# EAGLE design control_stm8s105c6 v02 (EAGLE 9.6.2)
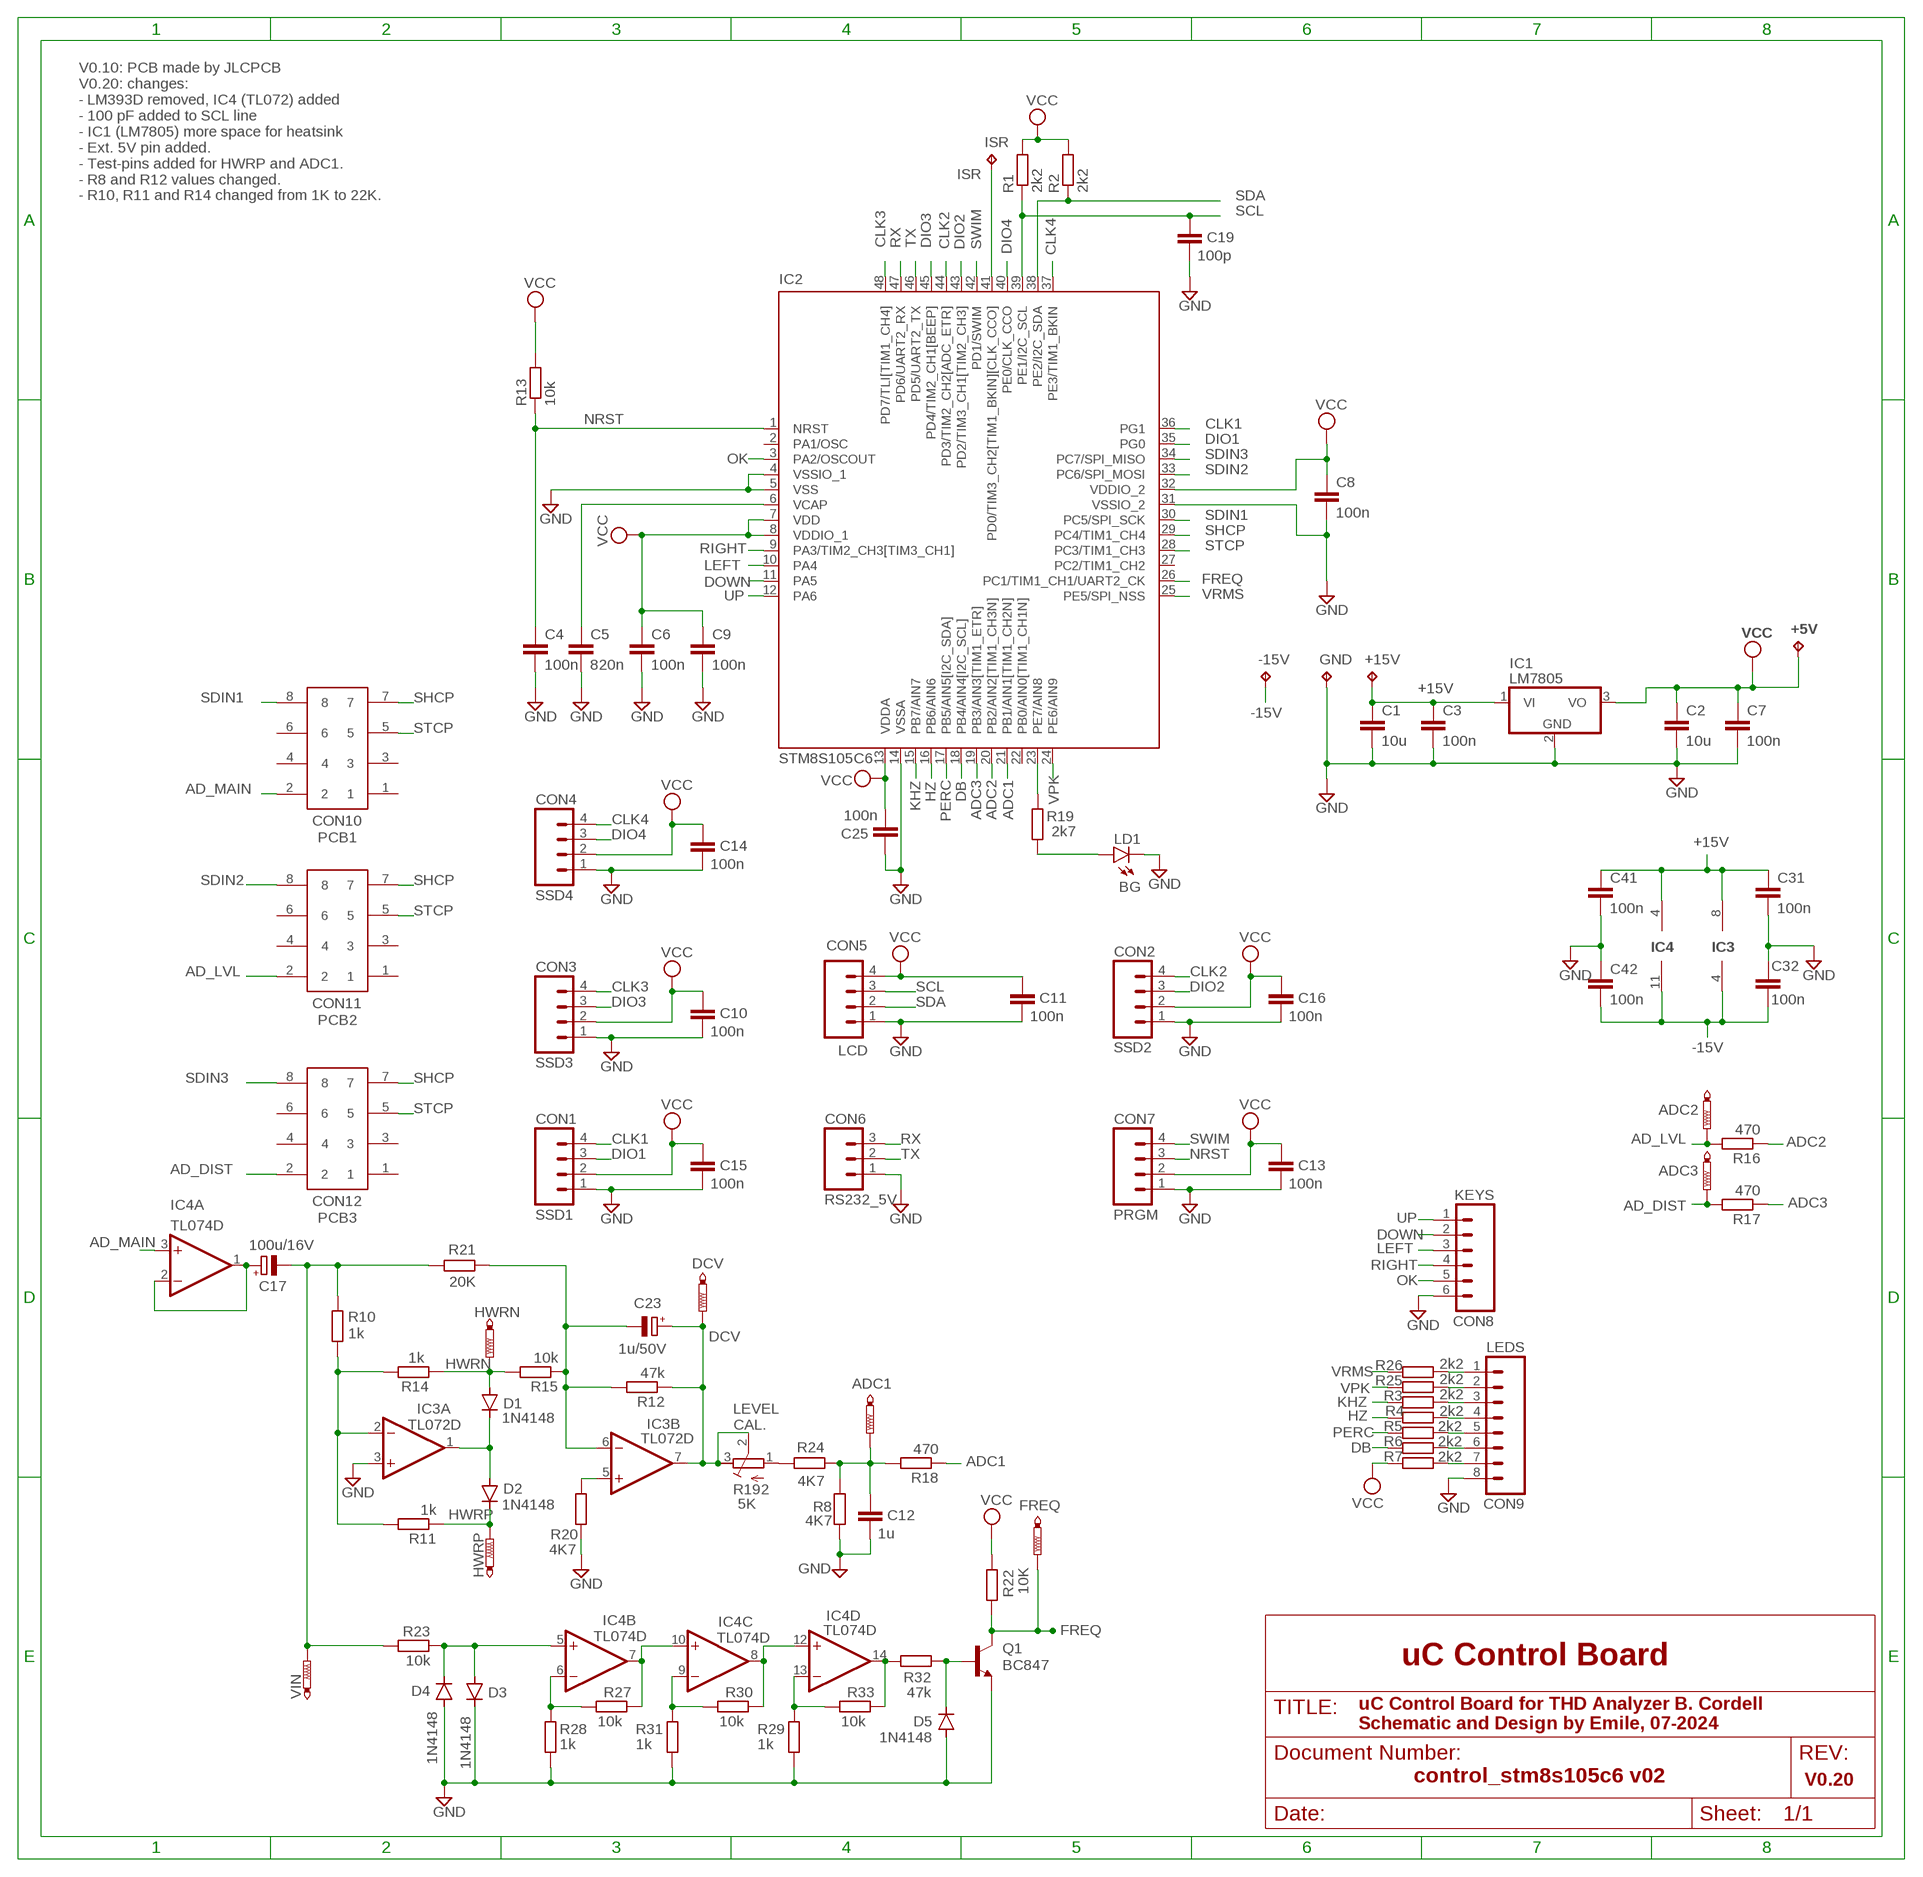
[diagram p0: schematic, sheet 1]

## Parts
+5V  TPPAD1-13Y  [P1-13Y]
+15V  TPPAD1-13Y  [P1-13Y]
-15V  TPPAD1-13Y  [P1-13Y]
ADC1  PTR1B2,54  [B2,54]
ADC2  PTR1B2,54  [B2,54]
ADC3  PTR1B2,54  [B2,54]
C1  10u  C-EUC1206  [C1206]
C2  10u  C-EUC1206  [C1206]
C3  100n  C-EUC1206  [C1206]
C4  100n  C-EUC1206K  [C1206K]
C5  820n  C-EUC1206K  [C1206K]
C6  100n  C-EUC1206K  [C1206K]
C7  100n  C-EUC1206  [C1206]
C8  100n  C-EUC1206K  [C1206K]
C9  100n  C-EUC1206K  [C1206K]
C10  100n  C-EUC1206  [C1206]
C11  100n  C-EUC1206  [C1206]
C12  1u  C-EUC1206  [C1206]
C13  100n  C-EUC1206  [C1206]
C14  100n  C-EUC1206  [C1206]
C15  100n  C-EUC1206  [C1206]
C16  100n  C-EUC1206  [C1206]
C17  100u/16V  CPOL-EUUD-6,3X8,8  [UD-6,3X5,8_NICHICON]
C19  100p  C-EUC1206  [C1206]
C23  1u/50V  CPOL-EUUD-4X5,8  [UD-4X5,8_NICHICON]
C25  100n  C-EUC1206  [C1206]
C31  100n  C-EUC1206  [C1206]
C32  100n  C-EUC1206  [C1206]
C41  100n  C-EUC1206  [C1206]
C42  100n  C-EUC1206  [C1206]
CON1  SSD1  M04  [04P]
CON2  SSD2  M04  [04P]
CON3  SSD3  M04  [04P]
CON4  SSD4  M04  [04P]
CON5  LCD  M04  [04P]
CON6  RS232_5V  M03  [03P]
CON7  PRGM  M04  [04P]
CON8  KEYS  M06  [06P]
CON9  LEDS  M08  [08P]
CON10  PCB1  61200821621  [61200821621]
CON11  PCB2  61200821621  [61200821621]
CON12  PCB3  61200821621  [61200821621]
D1  1N4148  D-SOD-80  [SOD80]
D2  1N4148  D-SOD-80  [SOD80]
D3  1N4148  D-SOD-80  [SOD80]
D4  1N4148  D-SOD-80  [SOD80]
D5  1N4148  D-SOD-80  [SOD80]
DCV  PTR1B2,54  [B2,54]
FREQ  PTR1B2,54  [B2,54]
GND  TPPAD1-13Y  [P1-13Y]
HWRN  PTR1B2,54  [B2,54]
HWRP  PTR1B2,54  [B2,54]
IC1  LM7805  7805TV  [TO220V]
IC2  STM8S105C6  STM8S105CV2  [LQFP48]
IC3  TL072D  [SO08]
IC4  TL074D  [SO14]
ISR  TPB2,54  [B2,54]
LD1  BG  LEDCHIPLED_1206  [CHIPLED_1206]
Q1  BC847  [SOT23]
R1  2k2  R-EU_R1206  [R1206]
R2  2k2  R-EU_R1206  [R1206]
R3  2k2  R-EU_M1206  [M1206]
R4  2k2  R-EU_M1206  [M1206]
R5  2k2  R-EU_M1206  [M1206]
R6  2k2  R-EU_M1206  [M1206]
R7  2k2  R-EU_M1206  [M1206]
R8  4K7  R-EU_R1206  [R1206]
R10  1k  R-EU_R1206  [R1206]
R11  1k  R-EU_R1206  [R1206]
R12  47k  R-EU_R1206  [R1206]
R13  10k  R-EU_R1206  [R1206]
R14  1k  R-EU_R1206  [R1206]
R15  10k  R-EU_R1206  [R1206]
R16  470  R-EU_R1206  [R1206]
R17  470  R-EU_R1206  [R1206]
R18  470  R-EU_R1206  [R1206]
R19  2k7  R-EU_M1206  [M1206]
R20  4K7  R-EU_R1206  [R1206]
R21  20K  R-EU_R1206  [R1206]
R22  10K  R-EU_R1206  [R1206]
R23  10k  R-EU_R1206  [R1206]
R24  4K7  R-EU_R1206  [R1206]
R25  2k2  R-EU_M1206  [M1206]
R26  2k2  R-EU_M1206  [M1206]
R27  10k  R-EU_R1206  [R1206]
R28  1k  R-EU_R1206  [R1206]
R29  1k  R-EU_R1206  [R1206]
R30  10k  R-EU_R1206  [R1206]
R31  1k  R-EU_R1206  [R1206]
R32  47k  R-EU_R1206  [R1206]
R33  10k  R-EU_R1206  [R1206]
R192  5K  R-TRIMM3296W  [RTRIM3296W]
VIN  PTR1B2,54  [B2,54]

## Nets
+15V: +15V.TP C1.1 C3.1 C31.1 C41.1 IC1.1(VI) IC3.8(P:V+) IC4.4(P:V+)
-15V: -15V.TP C32.2 C42.2 IC3.4(P:V-) IC4.11(P:V-)
AD_DIST: ADC3.TP CON12.2 R17.2
AD_LVL: ADC2.TP CON11.2 R16.2
AD_MAIN: CON10.2 IC4.3(A:+IN)
ADC1: IC2.21(PB1/AIN1[TIM1_CH2N]) R18.1
ADC2: IC2.20(PB2/AIN2[TIM1_CH3N]) R16.1
ADC3: IC2.19(PB3/AIN3[TIM1_ETR]) R17.1
CLK1: CON1.4 IC2.36(PG1)
CLK2: CON2.4 IC2.44(PD3/TIM2_CH2[ADC_ETR])
CLK3: CON3.4 IC2.48(PD7/TLI[TIM1_CH4])
CLK4: CON4.4 IC2.37(PE3/TIM1_BKIN)
DB: IC2.18(PB4/AIN4[I2C_SCL]) R6.1
DCV: C23.+ DCV.TP IC3.7(B:OUT) R12.1 R192.2(S) R192.3(E)
DIO1: CON1.3 IC2.35(PG0)
DIO2: CON2.3 IC2.43(PD2/TIM3_CH1[TIM2_CH3])
DIO3: CON3.3 IC2.45(PD4/TIM2_CH1[BEEP])
DIO4: CON4.3 IC2.40(PE0/CLK_CCO)
DOWN: CON8.2 IC2.11(PA5)
FREQ: FREQ.TP IC2.26(PC1/TIM1_CH1/UART2_CK) Q1.3(C) R22.1
GND: C1.2 C2.2 C3.2 C4.2 C5.2 C6.2 C7.2 C8.2 C9.2 C10.2 C11.2 C12.2 C13.2 C14.2 C15.2 C16.2 C19.2 C25.1 C31.2 C32.1 C41.2 C42.1 CON1.1 CON2.1 CON3.1 CON4.1 CON5.1 CON6.1 CON7.1 CON8.6 CON9.8 D3.1(C) D4.2(A) D5.2(A) GND.TP IC1.2(GND) IC2.4(VSSIO_1) IC2.5(VSS) IC2.14(VSSA) IC2.31(VSSIO_2) IC3.3(A:+IN) LD1.C Q1.2(E) R8.1 R20.2 R28.2 R29.2 R31.2
HWRN: D1.2(A) HWRN.TP R14.1 R15.2
HWRP: D2.1(C) HWRP.TP R11.1
HZ: IC2.16(PB6/AIN6) R4.1
ISR: IC2.41(PD0/TIM3_CH2[TIM1_BKIN][CLK_CCO]) ISR.TP
KHZ: IC2.15(PB7/AIN7) R3.1
LEFT: CON8.3 IC2.10(PA4)
N$1: CON9.3 R3.2
N$2: ADC1.TP C12.1 R8.2 R18.2 R24.1
N$3: CON9.1 R26.2
N$4: R24.2 R192.1(A)
N$5: CON9.4 R4.2
N$6: CON9.5 R5.2
N$7: CON9.6 R6.2
N$8: CON9.7 R7.2
N$9: CON9.2 R25.2
N$10: IC3.2(A:-IN) R10.2 R11.2 R14.2
N$11: C23.- IC3.6(B:-IN) R12.2 R15.1 R21.1
N$12: IC3.5(B:+IN) R20.1
N$13: IC2.23(PE7/AIN8) R19.2
N$14: LD1.A R19.1
N$16: D1.1(C) D2.2(A) IC3.1(A:OUT)
N$17: C17.+ IC4.1(A:OUT) IC4.2(A:-IN)
N$19: IC4.6(B:-IN) R27.2 R28.1
N$20: D3.2(A) D4.1(C) IC4.5(B:+IN) R23.2
N$21: IC4.7(B:OUT) IC4.10(C:+IN) R27.1
N$22: IC4.9(C:-IN) R30.2 R31.1
N$23: IC4.8(C:OUT) IC4.12(D:+IN) R30.1
N$24: IC4.13(D:-IN) R29.1 R33.2
N$25: D5.1(C) Q1.1(B) R32.2
N$26: IC4.14(D:OUT) R32.1 R33.1
NRST: C4.1 CON7.3 IC2.1(NRST) R13.1
OK: CON8.5 IC2.3(PA2/OSCOUT)
PERC: IC2.17(PB5/AIN5[I2C_SDA]) R5.1
RIGHT: CON8.4 IC2.9(PA3/TIM2_CH3[TIM3_CH1])
RX: CON6.3 IC2.47(PD6/UART2_RX)
SCL: C19.1 CON5.3 IC2.39(PE1/I2C_SCL) R1.1
SDA: CON5.2 IC2.38(PE2/I2C_SDA) R2.1
SDIN1: CON10.8 IC2.30(PC5/SPI_SCK)
SDIN2: CON11.8 IC2.33(PC6/SPI_MOSI)
SDIN3: CON12.8 IC2.34(PC7/SPI_MISO)
SHCP: CON10.7 CON11.7 CON12.7 IC2.29(PC4/TIM1_CH4)
STCP: CON10.5 CON11.5 CON12.5 IC2.28(PC3/TIM1_CH3)
SWIM: CON7.4 IC2.42(PD1/SWIM)
TX: CON6.2 IC2.46(PD5/UART2_TX)
UP: CON8.1 IC2.12(PA6)
VCAP: C5.1 IC2.6(VCAP)
VCC: +5V.TP C2.1 C6.1 C7.1 C8.1 C9.1 C10.1 C11.1 C13.1 C14.1 C15.1 C16.1 C25.2 CON1.2 CON2.2 CON3.2 CON4.2 CON5.4 CON7.2 IC1.3(VO) IC2.7(VDD) IC2.8(VDDIO_1) IC2.13(VDDA) IC2.32(VDDIO_2) R1.2 R2.2 R7.1 R13.2 R22.2
VIN: C17.- R10.1 R21.2 R23.1 VIN.TP
VPK: IC2.24(PE6/AIN9) R25.1
VRMS: IC2.25(PE5/SPI_NSS) R26.1
Unconnected: CON10.1 CON10.3 CON10.4 CON10.6 CON11.1 CON11.3 CON11.4 CON11.6 CON12.1 CON12.3 CON12.4 CON12.6 IC2.2(PA1/OSC) IC2.22(PB0/AIN0[TIM1_CH1N]) IC2.27(PC2/TIM1_CH2)

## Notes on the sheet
- V0.10: PCB made by JLCPCB
  V0.20: changes:
  - LM393D removed, IC4 (TL072) added
  - 100 pF added to SCL line
  - IC1 (LM7805) more space for heatsink
  - Ext. 5V pin added.
  - Test-pins added for HWRP and ADC1.
  - R8 and R12 values changed.
  - R10, R11 and R14 changed from 1K to 22K.
- IC4 | IC3
- LEVEL
  CAL.
- uC Control Board
- uC Control Board for THD Analyzer B. Cordell
  Schematic and Design by Emile, 07-2024
- V0.20

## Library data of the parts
+5V +15V -15V GND ISR = testpad:TP: Test pad
ADC1-ADC3 DCV FREQ HWRN HWRP VIN = testpad:PTR1: TEST PIN
C1-C16 C19 C25 C31 C32 C41 C42 = rcl:C-EU: CAPACITOR, European symbol
C17 C23 = rcl:CPOL-EU: POLARIZED CAPACITOR, European symbol; SPICEPREFIX: C
CON1-CON5 CON7 = con-amp-quick:M04: AMP QUICK CONNECTOR; OC_FARNELL: unknown; OC_NEWARK: unknown
CON6 = con-amp-quick:M03: AMP QUICK CONNECTOR; OC_FARNELL: unknown; OC_NEWARK: unknown
CON8 = con-amp-quick:M06: AMP QUICK CONNECTOR; OC_FARNELL: unknown; OC_NEWARK: unknown
CON9 = con-amp-quick:M08: AMP QUICK CONNECTOR; OC_FARNELL: unknown; OC_NEWARK: unknown
CON10-CON12 = Wurth_Elektronik_Electromechanic_Wire_to_Board_Connectors_rev16a:61200821621: WR-BHD 2.54mm Male Box Header, 8 Pins=>Code : Con_WTB_BHD_2.54_Male_THT_WS_61200821621 Details see: http://katalog.we-online.de/en/em/612_0xx_216_21 Created 2014-06-04, Karrer Zheng 2014 (C) Würth Elektronik
D1-D5 = semicon-smd-ipc:D-: DIODE
IC1 = linear:78*: Positive VOLTAGE REGULATOR Source: http://cache.national.com/ds/LM/LM78L05.pdf http://www.fairchildsemi.com/ds/LM/LM7805.pdf
IC2 = emile:STM8S105C: Access line, 16 MHz STM8S 8-bit MCU up to 32 Kbytes Flash, integrated EEPROM,10-bit ADC, timers, UART, SPI, I²C Source: Data sheet
IC3 = linear:TL072: OP AMP
IC4 = linear:TL074: OP AMP
LD1 = led:LED: LED
Q1 = transistor:BC847: NPN TRANSISTOR
R1-R8 R10-R33 = rcl:R-EU_: RESISTOR, European symbol
R192 = rcl:R-TRIMM: Trimm resistor; SPICEMODEL: X; SPICEPREFIXL: POT

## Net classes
1 power: width 0.254 mm

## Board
2024-07-10 PCB Made by JLCPCB.
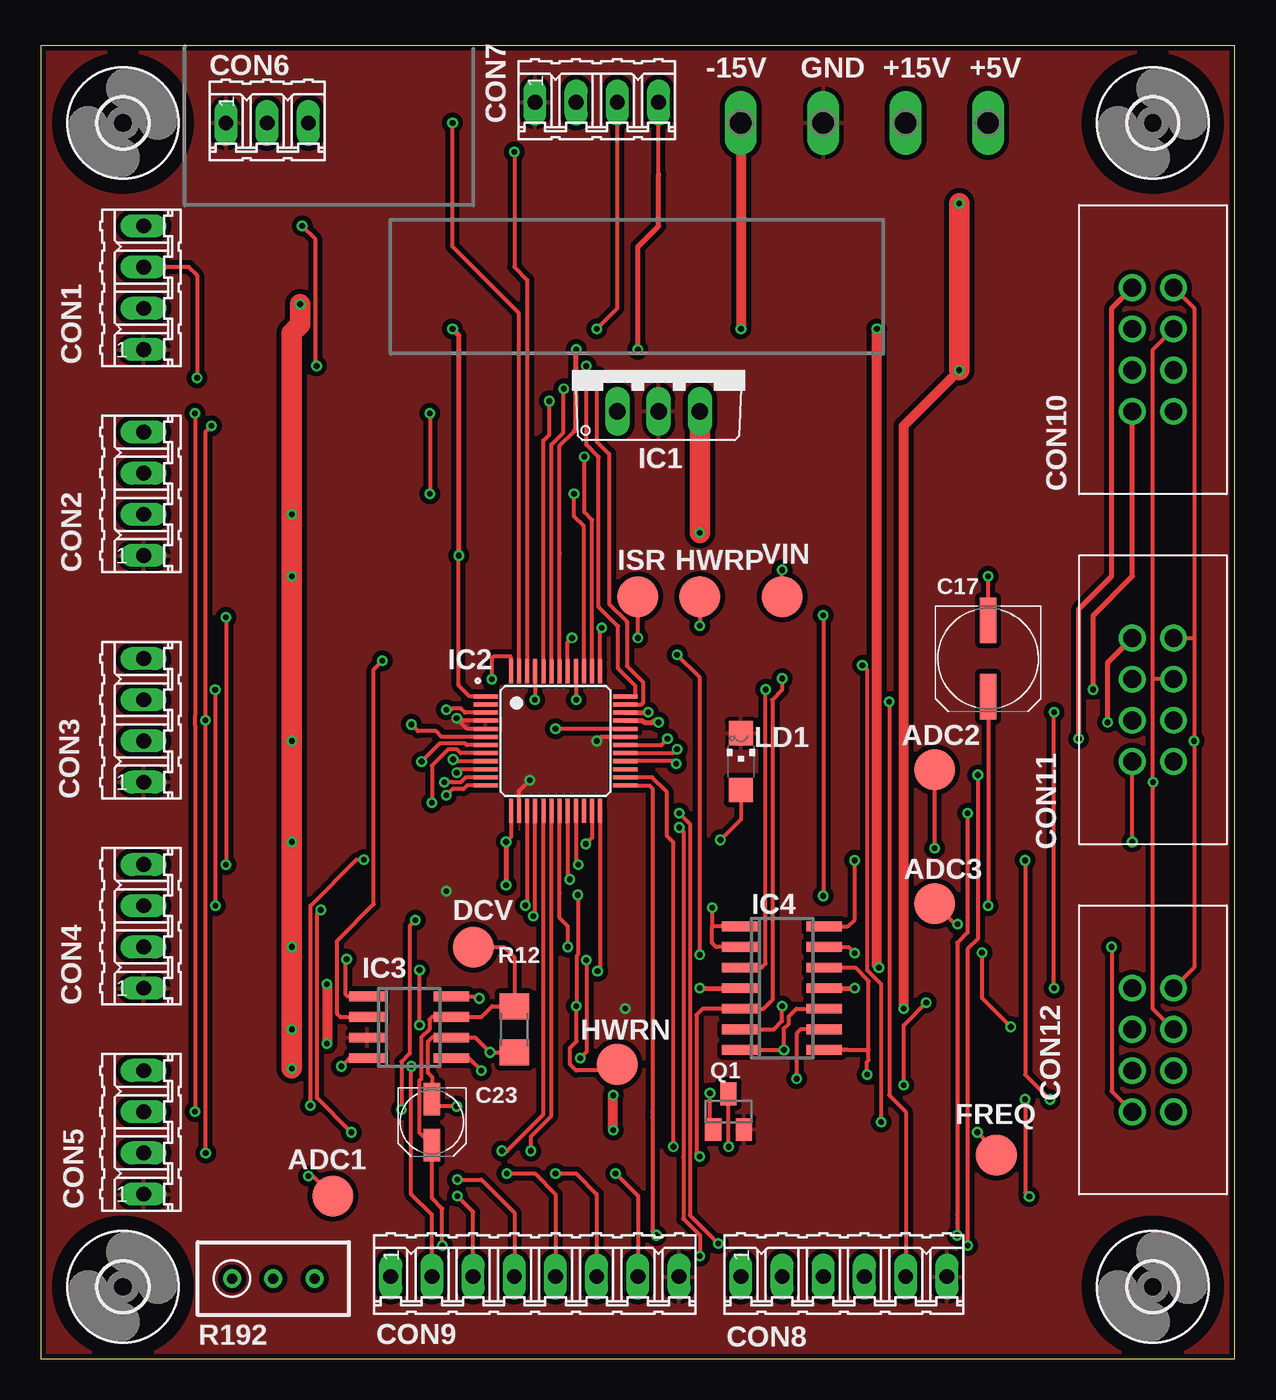
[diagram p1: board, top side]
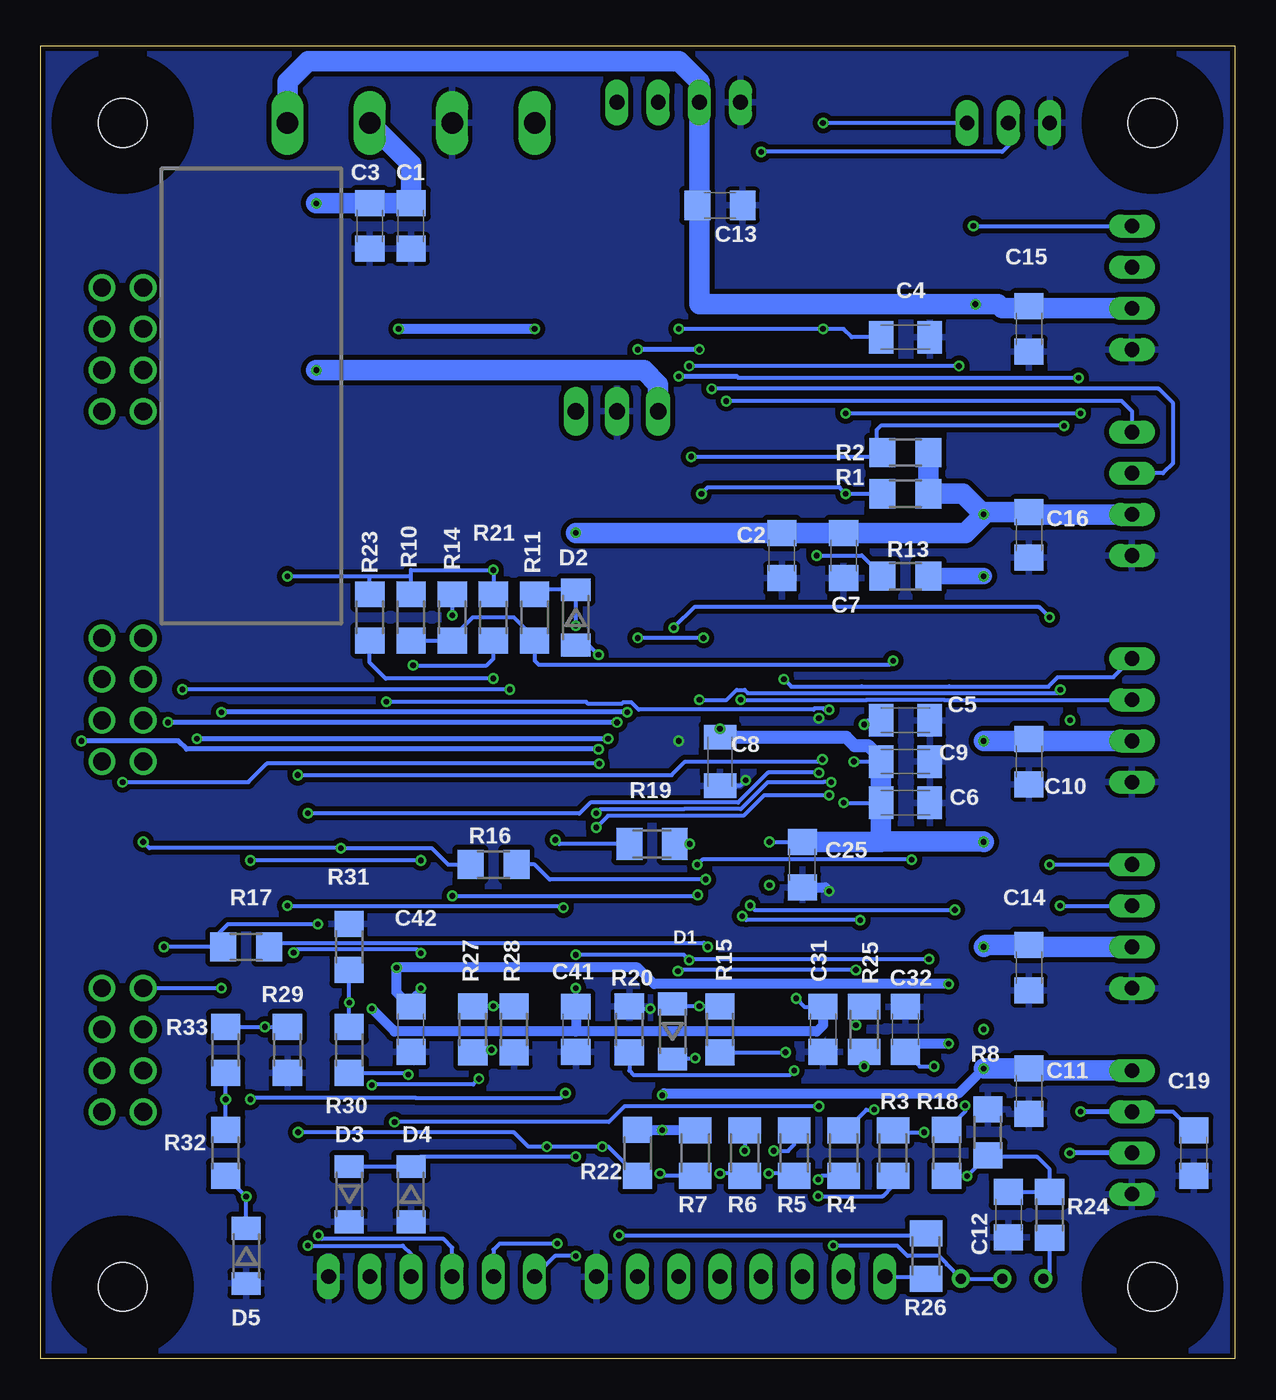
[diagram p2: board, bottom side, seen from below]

Size 73.64 x 80.95 mm. Coordinates in mm from the lower left corner, seen from the top.
Outline: 0,0 73.64,0 73.64,80.95 0,80.95 0,0
Copper layers (1*16): Top 0.035mm / dielectric 1.5mm / Bottom 0.035mm
Design rules "ITEADstudio_DRC for Eagle v6": minimum track width 6mil, minimum drill 12mil, track to track 6mil, track to pad 6mil, pad to pad 6mil, via to via 6mil, smd to smd 0mil, copper to edge 10mil, drill to drill 10mil, minimum pad ring 10mil, minimum via ring 6mil, stop-mask expansion 2mil, vias tented up to drill 100mil, thermal gap 10mil

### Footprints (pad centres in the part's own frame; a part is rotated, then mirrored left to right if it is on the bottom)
P1-13Y = drill 1.321 pad 1.905 long: TP 0,0
B2,54 = smd 2.54 x 2.54: TP 0,0
C1206 = smd 1.6 x 1.8: 1 -1.4,0; 2 1.4,0
C1206K = smd 1.5 x 2: 1 -1.5,0; 2 1.5,0
UD-6,3X5,8_NICHICON = smd 2.8 x 1: + 2.35,0; - -2.35,0
UD-4X5,8_NICHICON = smd 2 x 1: + 1.425,0; - -1.425,0
04P = drill 0.914 long: 1 -3.81,0; 2 -1.27,0; 3 1.27,0; 4 3.81,0
03P = drill 0.914 long: 1 -2.54,0; 2 0,0; 3 2.54,0
06P = drill 0.914 long: 1 -6.35,0; 2 -3.81,0; 3 -1.27,0; 4 1.27,0; 5 3.81,0; 6 6.35,0
08P = drill 0.914 long: 1 -8.89,0; 2 -6.35,0; 3 -3.81,0; 4 -1.27,0; 5 1.27,0; 6 3.81,0; 7 6.35,0; 8 8.89,0
61200821621 = drill 1.1: 1 -2.54,-1.27; 2 -2.54,1.27; 3 0,-1.27; 4 0,1.27; 5 2.54,-1.27; 6 2.54,1.27; 7 5.08,-1.27; 8 5.08,1.27
SOD80 = smd 1.4 x 1.8: 1 -1.7,0; 2 1.7,0
TO220V = drill 1.016 long: 1 -2.54,-2.54; 2 0,-2.54; 3 2.54,-2.54
LQFP48 = smd 1.5 x 0.25: 1 -4.3,2.75; 2 -4.3,2.25; 3 -4.3,1.75; 4 -4.3,1.25; 5 -4.3,0.75; 6 -4.3,0.25; 7 -4.3,-0.25; 8 -4.3,-0.75; 9 -4.3,-1.25; 10 -4.3,-1.75; 11 -4.3,-2.25; 12 -4.3,-2.75; 25 4.3,-2.75; 26 4.3,-2.25; 27 4.3,-1.75; 28 4.3,-1.25; 29 4.3,-0.75; 30 4.3,-0.25; 31 4.3,0.25; 32 4.3,0.75; 33 4.3,1.25; 34 4.3,1.75; 35 4.3,2.25; 36 4.3,2.75 | smd 0.25 x 1.5: 13 -2.75,-4.3; 14 -2.25,-4.3; 15 -1.75,-4.3; 16 -1.25,-4.3; 17 -0.75,-4.3; 18 -0.25,-4.3; 19 0.25,-4.3; 20 0.75,-4.3; 21 1.25,-4.3; 22 1.75,-4.3; 23 2.25,-4.3; 24 2.75,-4.3; 37 2.75,4.3; 38 2.25,4.3; 39 1.75,4.3; 40 1.25,4.3; 41 0.75,4.3; 42 0.25,4.3; 43 -0.25,4.3; 44 -0.75,4.3; 45 -1.25,4.3; 46 -1.75,4.3; 47 -2.25,4.3; 48 -2.75,4.3
SO08 = smd 0.6 x 2.2: 1 -1.905,-2.6; 2 -0.635,-2.6; 3 0.635,-2.6; 4 1.905,-2.6; 5 1.905,2.6; 6 0.635,2.6; 7 -0.635,2.6; 8 -1.905,2.6
SO14 = smd 0.6 x 2.2: 1 -3.81,-2.6; 2 -2.54,-2.6; 3 -1.27,-2.6; 4 0,-2.6; 5 1.27,-2.6; 6 2.54,-2.6; 7 3.81,-2.6; 8 3.81,2.6; 9 2.54,2.6; 10 1.27,2.6; 11 0,2.6; 12 -1.27,2.6; 13 -2.54,2.6; 14 -3.81,2.6
CHIPLED_1206 = smd 1.5 x 1.5: A 0,-1.75; C 0,1.75
SOT23 = smd 1 x 1.4: 1 -0.95,-1.1; 2 0.95,-1.1; 3 0,1.1
R1206 = smd 1.6 x 1.803: 1 -1.422,0; 2 1.422,0
M1206 = smd 1.6 x 2: 1 -1.4,0; 2 1.4,0
RTRIM3296W = drill 0.61: 1 0,-2.54; 2 0,0; 3 0,2.54
3,0 = hole 3: 0,0

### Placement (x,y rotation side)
+5V  58.42,76.2 0 top
+15V  53.34,76.2 0 top
-15V  43.18,76.2 0 top
ADC1  18.03,10.03 0 top
ADC2  55.12,36.32 0 top
ADC3  55.12,28.07 0 top
C1  50.8,69.85 270 bottom
C2  27.94,49.53 270 bottom
C3  53.34,69.85 270 bottom
C4  20.32,62.99 0 bottom
C5  20.32,39.37 0 bottom
C6  20.32,36.83 0 bottom
C7  24.13,49.53 270 bottom
C8  31.75,36.83 270 bottom
C9  20.32,34.29 0 bottom
C10  12.7,36.83 270 bottom
C11  12.7,16.51 270 bottom
C12  13.97,8.89 270 bottom
C13  31.75,71.12 0 bottom
C14  12.7,24.13 270 bottom
C15  12.7,63.5 270 bottom
C16  12.7,50.8 270 bottom
C17  58.42,43.18 270 top
C19  2.54,12.7 270 bottom
C23  24.13,14.61 270 top
C25  26.67,30.48 90 bottom
C31  25.4,20.32 270 bottom
C32  20.32,20.32 270 bottom
C41  40.64,20.32 270 bottom
C42  50.8,20.32 90 bottom
CON1  6.35,66.04 90 top
CON2  6.35,53.34 90 top
CON3  6.35,39.37 90 top
CON4  6.35,26.67 90 top
CON5  6.35,13.97 90 top
CON6  13.97,76.2 0 top
CON7  34.29,77.47 0 top
CON8  49.53,5.08 0 top
CON9  30.48,5.08 0 top
CON10  68.58,60.96 90 top
CON11  68.58,39.37 90 top
CON12  68.58,17.78 90 top
D1  34.67,20.19 90 bottom
D2  40.64,45.72 270 bottom
D3  54.61,10.16 90 bottom
D4  50.8,10.16 270 bottom
D5  60.96,6.35 270 bottom
DCV  26.67,25.4 0 top
FREQ  58.93,12.57 0 top
GND  48.26,76.2 0 top
HWRN  35.56,18.16 0 top
HWRP  40.64,46.99 0 top
IC1  38.1,60.96 0 top
IC2  31.75,38.1 0 top
IC3  22.73,20.45 270 top
IC4  45.72,22.86 270 top
ISR  36.83,46.99 0 top
LD1  43.18,36.83 0 top
Q1  42.42,15.24 0 top
R1  20.32,53.34 0 bottom
R2  20.32,55.88 0 bottom
R3  21.08,12.7 270 bottom
R4  24.13,12.7 270 bottom
R5  27.18,12.7 270 bottom
R6  30.23,12.7 270 bottom
R7  33.27,12.7 270 bottom
R8  15.24,13.97 270 bottom
R10  50.8,45.72 270 bottom
R11  43.18,45.72 270 bottom
R12  29.21,20.32 270 top
R13  20.32,48.26 0 bottom
R14  48.26,45.72 270 bottom
R15  31.75,20.32 90 bottom
R16  45.72,30.48 180 bottom
R17  60.96,25.4 180 bottom
R18  17.78,12.7 270 bottom
R19  35.94,31.75 0 bottom
R20  37.34,20.32 90 bottom
R21  45.72,45.72 90 bottom
R22  36.83,12.7 90 bottom
R23  53.34,45.72 270 bottom
R24  11.43,8.89 270 bottom
R25  22.86,20.32 270 bottom
R26  19.05,6.35 270 bottom
R27  46.99,20.32 90 bottom
R28  44.45,20.32 270 bottom
R29  58.42,19.05 270 bottom
R30  54.61,19.05 90 bottom
R31  54.61,25.4 90 bottom
R32  62.23,12.7 270 bottom
R33  62.23,19.05 90 bottom
R192  14.35,4.95 270 top
U$1  [3,0]  5.08,76.2 0 top
U$2  [3,0]  5.08,4.45 0 top
U$3  [3,0]  68.58,4.45 0 top
U$4  [3,0]  68.58,76.2 0 top
VIN  45.72,46.99 0 top

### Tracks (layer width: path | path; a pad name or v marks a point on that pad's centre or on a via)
+15V  (via drill 0.35)
  Top 0.254: IC3.8 26.92,22.35 v27.05,22.23
  Top 0.305: v40.64,22.86 IC4.4
  Top 0.61: v53.21,21.59 53.21,57.53 v56.64,60.96
  Top 1.27: v56.64,71.25 v56.64,60.96
  Bottom 0.254: v27.05,22.23 26.55,21.72 C31.1
  Bottom 0.305: C41.1 v40.64,22.86
  Bottom 0.61: C31.1 25.4,20.57 25.78,20.19 40.64,20.19 | 40.64,20.19 51.82,20.19 v53.21,21.59 | C41.1 40.64,20.19
  Bottom 1.27: +15V.TP 50.8,73.66 C1.1 C3.1 v56.64,71.25 | IC1.1 35.56,60.07 36.45,60.96 v56.64,60.96
-15V  (via drill 0.35)
  Top 0.254: v18.54,18.03 19.05,18.54 IC3.4
  Top 0.305: IC4.11 v50.19,22.86
  Top 0.61: v51.56,63.5 51.54,63.48 51.54,24.28 v51.69,24.13 | -15V.TP v43.18,63.5 | v17.65,23.11 v17.65,19.43
  Bottom 0.254: C32.2 19.43,18.03 v18.54,18.03
  Bottom 0.305: v50.19,22.86 50.8,22.25 C42.2
  Bottom 0.61: v17.65,23.11 35.81,23.11 36.83,24.13 v51.69,24.13 51.69,22.61 C42.2 | v43.18,63.5 v51.56,63.5 | v17.65,19.43 19.81,19.43 C32.2
AD_DIST  (via drill 0.35)
  Top 0.254: v66.04,25.4 66.04,16.51 CON12.2 | ADC3.TP 56.39,26.8 v56.54,26.8
  Bottom 0.254: R17.2 62.61,25.4 | 62.61,25.4 v66.04,25.4 | v56.54,26.8 62.1,26.8 62.61,26.29 62.61,25.4
AD_LVL  (via drill 0.35)
  Top 0.254: v67.31,31.88 CON11.2 | ADC2.TP v55.12,31.5
  Bottom 0.254: R16.2 48.51,30.48 49.53,31.5 v55.12,31.5 66.93,31.5 v67.31,31.88
AD_MAIN  (via drill 0.35)
  Top 0.254: IC4.3 44.45,24.13 44.7,24.38 v44.7,41.27
  Top 0.305: v64.9,41.27 64.9,45.85 67.31,48.26 CON10.2
  Bottom 0.254: v44.7,41.27 v64.9,41.27
ADC1  (via drill 0.35)
  Top 0.254: IC2.21 33,30.63 v33.15,30.48 | v16.64,15.62 16.64,27.94 19.48,30.79 v19.94,30.79
  Bottom 0.254: v16.64,15.62 16.64,15.27 R18.1 | v19.94,30.79 32.84,30.79 v33.15,30.48
ADC2  (via drill 0.35)
  Top 0.254: IC2.20 32.5,29.69 v32.63,29.56
  Bottom 0.254: v32.63,29.56 42.26,29.56 43.18,30.48 R16.1
ADC3  (via drill 0.35)
  Top 0.254: IC2.19 32,28.71 32,28.7 32,27.18 32.51,26.67 v32.51,25.4
  Bottom 0.254: R17.1 59.28,25.65 32.77,25.65 v32.51,25.4
CLK1  (via drill 0.35)
  Top 0.254: v17.02,61.21 17.02,61.09 16.95,61.15 16.95,69.03 v16.13,69.85 | IC2.36 36.61,40.85 36.61,40.86 36.67,40.92 36.67,41.5 35.61,42.57 35.61,45.16 34.41,46.37 34.41,55.61 33.66,56.36 v33.66,61.21
  Bottom 0.254: v17.02,61.21 v33.66,61.21 | v16.13,69.85 CON1.4
CLK2  (via drill 0.35)
  Top 0.254: IC2.44 31,56.63 31.37,57 v31.37,59.05
  Bottom 0.254: v31.37,59.05 6.99,59.05 6.35,58.42 CON2.4
CLK3  (via drill 0.35)
  Top 0.254: IC2.48 29,43.26 28.96,43.31 27.94,43.31 27.81,43.18 v27.81,41.91
  Bottom 0.254: v27.81,41.91 27.36,41.45 23.03,41.45 23.02,41.46 17.62,41.46 17.61,41.45 11.51,41.45 10.92,42.04 7.49,42.04 CON3.4
CLK4  (via drill 0.35)
  Top 0.254: IC2.37 34.5,44.98 v34.61,45.09 | v11.43,45.72 v11.43,30.48
  Bottom 0.254: v11.43,30.48 CON4.4 | v11.43,45.72 12.06,46.35 33.34,46.35 v34.61,45.09
DB  (via drill 0.35)
  Top 0.254: IC2.18 31.5,14.99 30.23,13.72 v30.23,12.83
  Bottom 0.254: R6.1 v30.23,12.83
DCV  (via drill 0.35)
  Top 0.254: v24.77,6.99 24.77,9.27 24.13,9.91 C23.+ 23.35,13.96 23.35,17.15 23.47,17.27 23.47,19.82 23.98,20.32 23.98,20.93 24.13,21.08 IC3.7 27.18,21.08 27.84,21.74 R12.1 29.21,24.77 28.57,25.4 DCV.TP
  Bottom 0.254: R192.2 R192.3 17.77,5.83 17.77,5.87 18.25,6.35 20.19,6.35 20.83,6.99 v24.77,6.99
DIO1  (via drill 0.35)
  Top 0.254: v9.65,60.48 9.65,66.8 9.14,67.31 CON1.3 | IC2.35 37.05,40.35 37.16,40.46 37.16,41.72 36.14,42.73 36.14,45.46 35.05,46.55 35.05,55.79 34.29,56.55 v34.29,60.58
  Bottom 0.254: v9.65,60.48 30.63,60.48 30.73,60.58
  Bottom 0.305: v34.29,60.58 30.73,60.58
DIO2  (via drill 0.35)
  Top 0.152: v32.26,59.82 32.23,59.79
  Top 0.254: 32.23,59.79 32.23,57.1 31.5,56.37 IC2.43
  Bottom 0.254: v32.26,59.82 4.7,59.82 3.81,58.93 3.81,55.24 4.45,54.61 CON2.3
DIO3  (via drill 0.35)
  Top 0.254: IC2.45 30.48,42.38 v30.48,40.64
  Bottom 0.254: v30.48,40.64 22.7,40.64 22.69,40.65 17.95,40.65 17.95,40.64 CON3.3
DIO4  (via drill 0.35)
  Top 0.254: IC2.40 33,40.66 v33.02,40.64 | v10.77,41.25 10.77,27.96 v10.79,27.94
  Bottom 0.254: v33.02,40.64 31.34,40.64 30.73,41.25 30.23,41.25 30.03,41.05 22.86,41.05 22.85,41.06 17.79,41.06 17.78,41.05 10.97,41.05 v10.77,41.25 | v10.79,27.94 CON4.3
DOWN  (via drill 0.35)
  Top 0.254: IC2.11 26.21,35.85 25.91,35.54 25.4,35.54 25.39,35.56 v24.89,35.56 | v39.37,33.66 40.03,32.99 40.03,8.86 v41.78,7.11
  Bottom 0.254: v24.89,35.56 25.39,35.56 25.4,35.54 28.82,35.54 30.47,33.89 33.98,33.89 33.99,33.88 39.14,33.88 v39.37,33.66 | v41.78,7.11 45.34,7.11 45.72,6.73 CON8.2
FREQ  (via drill 0.35)
  Top 0.254: IC2.26 37.71,35.85 38.61,34.95 38.61,32.26 39.02,31.85 v39.02,13.08 | v42.42,13.08 Q1.3 | v57.76,13.97 58.93,12.8 FREQ.TP
  Bottom 0.254: R22.1 38.63,13.08 v39.02,13.08 v42.42,13.08 43.56,13.08 44.45,13.97 v57.76,13.97
GND  (via drill 0.35)
  Top 0.254: IC2.31 34.54,38.35 v34.29,38.1 | IC2.4 25.8,39.35 v25.65,39.5 26.3,38.85 IC2.5 | IC2.14 29.5,35.02 v30.17,35.69
  Bottom 0.254: v30.17,35.69 30.52,35.33 C8.2 | R20.2 37.19,21.59 v36.05,21.59
  Bottom 0.61: C25.1 25.27,29.08 v25.02,28.83
  pour Bottom (isolate 0.305): 0,0 0,81.28 73.66,81.28 73.66,0
  pour Top (isolate 0.305): 0,0 0,81.28 73.66,81.28 73.66,0
HWRN  (via drill 0.35)
  Top 0.254: v48.26,45.85 v48.26,28.55 | v33.13,28.6 33.13,24.92 33.05,24.84 33.05,21.77 | 33.05,21.77 v33.02,21.74 | HWRN.TP 35.18,17.78 33.02,17.78 32.64,18.16 32.64,19.18 33.05,19.59 33.05,21.77
  Bottom 0.254: R15.2 v33.02,21.74 34.52,21.74 D1.2 | R14.1 v48.26,45.85 | v48.26,28.55 33.19,28.55 v33.13,28.6
HWRP  (via drill 0.35)
  Top 0.254: HWRP.TP v40.64,45.2
  Bottom 0.254: R11.1 42.9,47.42 D2.1 v40.64,45.2
HZ  (via drill 0.35)
  Top 0.254: v30.38,27.3 30.5,27.42 IC2.16 | v22.25,15.37 22.25,18.32 22.76,18.82 22.76,26.7 v23.11,27.05
  Bottom 0.254: R4.1 24,14.1 22.73,15.37 v22.25,15.37 | v23.11,27.05 30.13,27.05 v30.38,27.3
ISR  (via drill 0.35)
  Top 0.254: IC2.41 32.5,44.18 v32.77,44.45 | v36.83,44.45 ISR.TP
  Bottom 0.254: v32.77,44.45 v36.83,44.45
KHZ  (via drill 0.35)
  Top 0.254: IC2.15 30,28.07 v29.89,27.96 | v19.16,13.97 17.04,16.09 17.04,27.46 v17.27,27.69
  Bottom 0.254: v29.89,27.96 29.62,27.68 v17.27,27.68 v17.27,27.69 | R3.1 20.95,13.97 v19.16,13.97
LEFT  (via drill 0.35)
  Top 0.254: IC2.10 25.85,36.35 v25.65,36.15 | v57.15,33.66 57.15,26.29 56.52,25.65 56.52,8.89 56.52,8.38 v56.52,7.62
  Bottom 0.254: v25.65,36.15 28.79,36.15 30.63,34.3 39.74,34.3 40.41,33.63 57.12,33.63 v57.15,33.66 | v56.52,7.62 56.29,7.39 48.79,7.39 48.26,6.86 CON8.3
N$1  (via drill 0.35)
  Top 0.254: v25.7,10.03 26.67,9.06 CON9.3
  Bottom 0.254: v25.7,10.03 21.72,10.03 21.08,10.67 R3.2
N$2  (via drill 0.35)
  Top 0.254: ADC1.TP 16.79,11.28 v16.51,11.28
  Bottom 0.254: R18.2 v16.51,11.28 R8.2 15.14,12.45 12.19,12.45 11.43,11.68 R24.1 11.45,10.29 C12.1
N$3
  Bottom 0.254: CON9.1 19.18,5.08 R26.2
N$4
  Bottom 0.254: R192.1 11.43,5.33 R24.2
N$5  (via drill 0.35)
  Top 0.254: v25.7,11.05 27.18,11.05 29.21,9.02 CON9.4
  Bottom 0.254: R4.2 25.45,11.3 v25.7,11.05
N$6  (via drill 0.35)
  Top 0.254: v28.75,11.43 30.48,11.43 31.75,10.16 CON9.5
  Bottom 0.254: R5.2 27.31,11.43 v28.75,11.43
N$7  (via drill 0.35)
  Top 0.254: v31.75,11.43 33.02,11.43 34.29,10.16 CON9.6
  Bottom 0.254: R6.2 30.36,11.43 v31.75,11.43
N$8  (via drill 0.35)
  Top 0.254: v35.45,11.43 36.83,10.05 CON9.7
  Bottom 0.254: R7.2 35.32,11.3 v35.45,11.43
N$9  (via drill 0.35)
  Top 0.254: CON9.2 24.13,8.89 22.86,10.16 v22.86,18.03
  Bottom 0.254: v22.86,18.03 R25.2
N$10  (via drill 0.35)
  Top 0.254: v21.08,43.05 20.55,42.52 20.55,28.04 18.26,25.75 18.26,21.31 18.49,21.08 IC3.2
  Bottom 0.254: R10.2 R14.2 48.26,44.45 46.99,45.72 44.45,45.72 43.18,44.45 R11.2 43.18,43.05 42.93,42.8 21.34,42.8 v21.08,43.05
N$11  (via drill 0.35)
  Top 0.254: v25.65,15.58 24.58,15.58 C23.- 24.13,17.4 23.88,17.65 23.88,19.56 24.13,19.81 IC3.6 26.8,19.81 v27.71,18.9 R12.2 | v50.67,42.77 50.95,42.48 50.95,23.98 51.82,23.11 v51.82,14.61
  Bottom 0.254: v51.82,14.61 38.61,14.61 37.64,15.58 v25.65,15.58 | v50.67,42.77 46.13,42.77 45.72,43.18 R21.1 | R15.1 v27.71,18.9
N$12  (via drill 0.35)
  Top 0.254: IC3.5 26.42,18.54 v27.18,17.78
  Bottom 0.254: R20.1 37.34,17.78 37.07,17.51 27.44,17.51 v27.18,17.78
N$13  (via drill 0.35)
  Top 0.254: IC2.23 34,32.14 v33.61,31.75
  Bottom 0.254: v33.61,31.75 R19.2
N$14  (via drill 0.35)
  Top 0.254: LD1.A 43.18,33.27 v41.91,32
  Bottom 0.254: R19.1 41.66,31.75 v41.91,32
N$16  (via drill 0.35)
  Top 0.254: v33.66,24.59 33.66,18.92 v33.27,18.54 | v40.64,24.91 40.64,42.01 v39.24,43.41 | IC3.1 18.92,22.35 18.8,22.48 18.8,24.57 v18.87,24.64
  Bottom 0.254: v18.87,24.64 33.6,24.64 v33.66,24.59 33.98,24.91 v40.64,24.91 | v33.27,18.54 33.32,18.49 D1.1 | v39.24,43.41 39.86,44.02 D2.2
N$17  (via drill 0.35)
  Top 0.254: IC4.2 41.66,25.4 41.4,25.65 41.4,26.67 | C17.+ v58.42,27.94 | v41.4,27.81 41.4,26.67 | IC4.1 41.4,26.67
  Bottom 0.254: v58.42,27.94 41.53,27.94 v41.4,27.81
N$19  (via drill 0.35)
  Top 0.254: IC4.6 45.21,20.32 45.72,20.83 v45.72,21.74
  Bottom 0.254: R28.1 v45.72,21.74 R27.2
N$20  (via drill 0.35)
  Top 0.254: v45.72,41.95 45.72,41.25 45.11,40.64 45.11,22.12 44.58,21.59 IC4.5 40.82,21.59 40.44,21.21 40.44,12.68 v40.64,12.47
  Bottom 0.254: D3.2 D4.1 50.19,12.47 v40.64,12.47 | v45.72,41.95 52.36,41.95 53.34,42.93 R23.2
N$21  (via drill 0.35)
  Top 0.254: IC4.7 v45.83,19.05 45.83,20.36 46.13,20.66 46.13,21.11 46.61,21.59 IC4.10
  Bottom 0.254: v45.83,19.05 46.84,19.05 R27.1
N$22  (via drill 0.35)
  Top 0.254: IC4.9 46.86,20.32 46.61,20.07 v46.61,17.27 | v53.21,16.89 53.21,20.57 v54.61,21.97
  Bottom 0.254: R30.2 v54.61,21.97 R31.1 | v46.61,17.27 46.96,16.92 53.19,16.92 v53.21,16.89
N$23  (via drill 0.35)
  Top 0.254: IC4.8 49.53,19.05 49.78,19.05 51.05,19.05 | IC4.12 50.23,24.13 51.05,23.3 51.05,19.05 | 51.05,19.05 51.05,18.41 50.95,18.32 v50.95,17.53
  Bottom 0.254: R30.1 51.06,17.63 v50.95,17.53
N$24  (via drill 0.35)
  Top 0.254: IC4.13 49.81,25.4 v50.19,25.02 | v58.04,25.05 58.04,22.25 v59.82,20.47
  Bottom 0.254: R33.2 v59.82,20.47 R29.1 | v50.19,25.02 50.42,25.25 57.84,25.25 v58.04,25.05
N$25  (via drill 0.35)
  Top 0.254: Q1.1 41.27,14.33 v41.27,16.38 | v60.71,16 60.71,10.26 v60.96,10.01
  Bottom 0.254: D5.1 v60.96,10.01 R32.2 | v60.71,16 60.61,16.1 50.8,16.1 50.55,16.1 41.56,16.1 v41.27,16.38
N$26  (via drill 0.35)
  Top 0.254: IC4.14 49.78,26.67 50.19,27.08 v50.19,30.73 | v60.71,30.73 60.71,17.53 v62.23,16
  Bottom 0.254: R32.1 v62.23,16 R33.1 | v50.19,30.73 v60.71,30.73
NRST  (via drill 0.35)
  Top 0.254: IC2.1 26.46,40.85 25.78,41.53 v25.78,49.53 | v34.29,63.5 35.56,64.77 CON7.3
  Top 0.305: v25.4,63.5 25.78,63.12 v25.78,49.53
  Bottom 0.254: v34.29,63.5 v25.4,63.5 24.13,63.5 23.62,62.99 C4.1 | v25.78,49.53 23.01,49.53 R13.1
OK  (via drill 0.35)
  Top 0.254: v25.02,40.03 25.33,40.03 25.4,40.1 25.91,40.1 26.16,39.85 IC2.3 | CON8.5 53.34,15.24 52.32,16.26 v52.32,40.51
  Bottom 0.254: v25.02,40.03 25.33,40.03 25.4,40.1 25.91,40.1 25.98,40.03 36.77,40.03 37.22,40.48 37.72,40.48 37.81,40.39 39.88,40.39 40,40.51 v52.32,40.51
PERC  (via drill 0.35)
  Top 0.254: IC2.17 30.99,33.79 30.99,15.05 28.76,12.83 v28.45,12.83
  Bottom 0.254: v28.45,12.83 27.56,12.83 27.18,13.21 R5.1
RIGHT  (via drill 0.35)
  Top 0.254: v25.43,36.96 25.54,36.85 IC2.9 | v57.78,36 57.78,25.91 57.15,25.27 v57.15,6.99
  Bottom 0.254: v57.78,36 34.74,36 33.91,36.83 25.56,36.83 v25.43,36.96 | v57.15,6.99 51.31,6.99 50.8,6.48 CON8.4
RX  (via drill 0.35)
  Top 0.254: IC2.47 29.5,64.48 25.4,68.58 v25.4,76.2
  Bottom 0.254: v25.4,76.2 CON6.3
SCL  (via drill 0.35)
  Top 0.254: v24,58.29 v24,53.34 | v9.53,15.24 9.53,39.08 9.5,39.1 9.5,39.64 9.53,39.66 v9.53,58.29 | IC2.39 33.5,51.34 32.89,51.94 v32.89,53.34
  Bottom 0.254: v9.53,58.29 v24,58.29 | R1.1 v24,53.34 24.38,53.72 32.51,53.72 v32.89,53.34 | C19.1 2.67,14.1 3.81,15.24 CON5.3
  Bottom 0.305: CON5.3 v9.53,15.24
SDA  (via drill 0.35)
  Top 0.254: v10.54,57.53 10.16,57.15 v10.16,39.37 10.18,39.35 v10.18,12.7 | v33.53,55.63 33.53,52.2 34,51.73 IC2.38
  Bottom 0.152: 22.23,55.63 21.86,55.99
  Bottom 0.254: v10.54,57.53 21.84,57.53 22.1,57.28 22.1,56.24 21.86,55.99 R2.1 | v33.53,55.63 22.23,55.63
  Bottom 0.305: CON5.2 v10.18,12.7
SDIN1  (via drill 0.35)
  Top 0.254: IC2.30 38.28,37.85 v38.65,38.23
  Top 0.305: v64.01,38.23 64.01,46.23 66.04,48.26 66.04,64.77 CON10.8
  Bottom 0.305: v38.65,38.23 v64.01,38.23
SDIN2  (via drill 0.35)
  Top 0.305: v38.1,39.24 37.99,39.35 37.84,39.35 37.73,39.24 37.21,39.24 37.1,39.35 IC2.33 | v65.79,39.24 65.79,42.93 CON11.8
  Bottom 0.305: v65.79,39.24 | v38.1,39.24 v65.79,39.24
SDIN3  (via drill 0.35)
  Top 0.254: v62.48,22.86 v62.48,39.88
  Top 0.305: IC2.34 37.31,39.85 37.34,39.88 v37.47,39.88
  Bottom 0.254: v62.48,22.86 CON12.8
  Bottom 0.305: v37.47,39.88 v62.48,39.88
SHCP  (via drill 0.35)
  Top 0.254: IC2.29 39,37.35 v39.24,37.59 | CON10.7 71.12,64.77 71.12,44.45 | 71.12,44.45 v71.12,38.1 71.12,24.13 CON12.7 | CON11.7 71.12,44.45
  Bottom 0.305: v39.24,37.59 64.65,37.59 65.15,38.1 v71.12,38.1
STCP  (via drill 0.35)
  Top 0.254: CON12.5 68.58,21.59 v68.58,35.56 68.58,41.91 | 68.58,41.91 68.58,62.23 CON10.5 | CON11.5 68.58,41.91 | v39.19,36.7 39.04,36.85 IC2.28
  Bottom 0.254: v39.19,36.7 59.69,36.7 60.83,35.56 v68.58,35.56
SWIM  (via drill 0.35)
  Top 0.254: IC2.42 32,49.65 32,49.66 32,56.3 32.92,57.21 | 38.1,73.03 CON7.4
  Top 0.305: 32.92,57.21 33.02,57.32 v33.02,62.23 | 38.1,73.03 38.1,69.85 36.83,68.58 v36.83,62.23
  Bottom 0.305: v33.02,62.23 v36.83,62.23
TX  (via drill 0.35)
  Top 0.254: IC2.46 30,66.52 29.21,67.31 v29.21,74.42
  Bottom 0.254: CON6.2 13.97,74.8 14.35,74.42 v29.21,74.42
UP  (via drill 0.35)
  Top 0.254: IC2.12 26.29,35.35 26.07,35.14 25.4,35.14 v25.02,34.75 | v39.37,32.77 39.62,32.51 39.62,12.45 39.62,8.64 40.64,7.62 v40.64,6.35
  Bottom 0.254: v25.02,34.75 29.03,34.75 30.31,33.48 38.66,33.48 v39.37,32.77 | v40.64,6.35 41.91,6.35 CON8.1
VCAP  (via drill 0.35)
  Top 0.254: IC2.6 25.4,38.35 25.28,38.35 24.74,38.35 24.38,38.71 23.27,38.71 v22.86,39.12
  Bottom 0.254: C5.1 22.61,39.37 v22.86,39.12
VCC  (via drill 0.35)
  Top 0.254: IC2.13 29,32.17 v28.7,31.88 | IC2.32 31.76,38.85 v31.75,38.86 | IC2.8 25.9,37.35 25.69,37.56 25.12,37.56 24.13,36.58 v24.13,34.29 | IC2.7 26.29,37.85 26.19,37.94 24.61,37.94 v23.5,36.83
  Top 0.305: v28.7,31.88 v28.7,29.21
  Top 0.61: v35.31,14.1 v35.31,16.26
  Top 1.27: v16,65.02 16,63.75 15.49,63.25 v15.49,52.07 v15.49,48.26 v15.49,38.1 v15.49,31.88 v15.49,25.4 v15.49,20.32 v15.49,17.91 | v40.64,50.93 IC1.3
  Bottom 0.254: v28.7,31.88 C25.2 | C8.1 v31.75,38.86 | v24.13,34.29 C9.1 | v23.5,36.83 C6.1
  Bottom 0.61: R7.1 v35.31,14.1 36.81,14.1 R22.2 | v35.31,16.26 35.18,16.38 17.02,16.38 v15.49,17.91
  Bottom 0.813: C8.1 23.98,38.33 23.46,37.81 22.61,37.81 21.82,37.02 C6.1
  Bottom 1.016: R13.2 v15.49,48.26
  Bottom 1.27: C11.1 | R2.2 R1.2 16.76,53.34 v15.49,52.07 | CON1.2 12.57,64.77 C15.1 12.83,64.77 14.35,64.77 14.61,65.02 v16,65.02 33.02,65.02 33.02,70.99 C13.1 33.02,71.25 CON7.2 33.02,78.74 34.29,80.01 57.15,80.01 58.42,78.74 +5V.TP | CON2.2 12.57,52.07 C16.1 15.36,52.2 v15.49,52.07 | CON3.2 12.57,38.1 C10.1 12.83,38.1 v15.49,38.1 | C6.1 C9.1 21.82,31.9 | 21.82,31.9 21.84,31.88 21.85,31.88 C25.2 | 21.82,31.9 15.52,31.9 v15.49,31.88 | v15.49,25.4 15.36,25.53 C14.1 12.57,25.4 CON4.2 | CON5.4 12.57,17.78 C11.1 | v15.49,17.91 C11.1 | v40.64,50.93 C2.1 C7.1 16.63,50.93 v15.49,52.07
VIN  (via drill 0.35)
  Top 0.254: C17.- v58.42,48.26 | VIN.TP v45.72,48.64
  Bottom 0.254: R21.2 v45.72,48.64 50.8,48.64 50.8,48.26 | v58.42,48.26 53.34,48.26 | 53.34,48.26 50.8,48.26 | R10.1 50.8,48.26 | R23.1 53.34,48.26
VPK  (via drill 0.35)
  Top 0.254: IC2.24 34.5,24.06 v34.34,23.9 | v23.37,20.57 v23.37,23.98
  Bottom 0.254: R25.1 23.37,21.21 v23.37,20.57 | v23.37,23.98 34.26,23.98 v34.34,23.9
VRMS  (via drill 0.35)
  Top 0.254: IC2.25 37.55,35.35 37.72,35.18 37.72,15.24 37.72,14.86 37.72,7.87 v37.97,7.62
  Bottom 0.254: v37.97,7.62 19.18,7.62 R26.1

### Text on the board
tDocu: GND / TX / RX | EXT. | GND | +5V | NRST | SWIM | THD Analyzer B. Cordell / Control Board V0.20 / PCB by Emile 07-2024 | CLK1 / DIO1 / VCC / GND | MAIN_OUT | CLK2 / DIO2 / VCC / GND | CLK3 / DIO3 / VCC / GND | LVL_IN | CLK4 / DIO4 / VCC / GND | DIST | VCC / SCL / SDA / GND | RMS | PK | kHz | Hz | % | dB | PWR | GND | UP | DOWN | LEFT | RIGHT | OK | GND
bDocu: THD Analyzer B. Cordell / Control Board V0.20 / PCB by Emile 07-2024 / Bottom-Layer

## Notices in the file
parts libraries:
Wurth_Elektronik_Electromechanic_Wire_to: Copyright: Würth Elektronik
